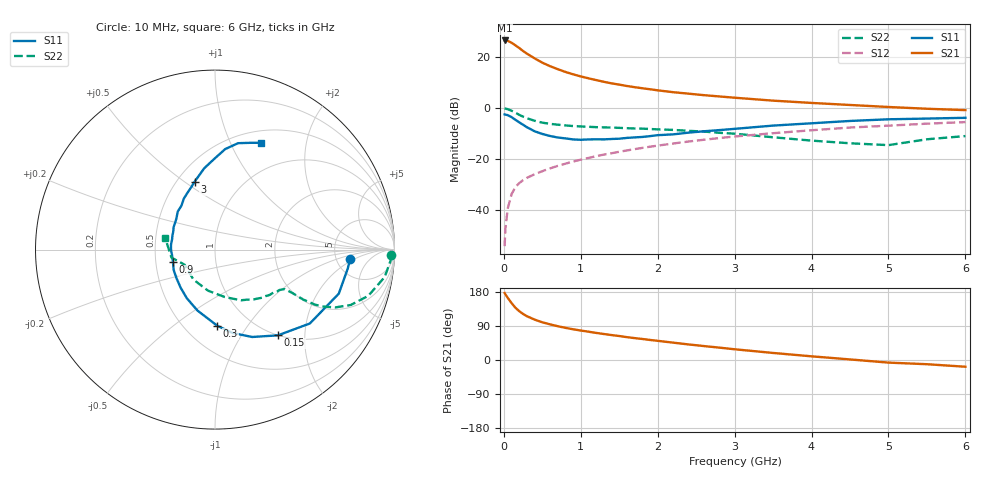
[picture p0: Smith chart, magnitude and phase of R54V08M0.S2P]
! SIEMENS Small Signal Semiconductors
! BFR183
! Si NPN RF Bipolar Junction Transistor in SOT23
! VCE = 4 V  IC = 8 mA
! Common Emitter S-Parameters:  May  1996
# GHz  S  MA  R  50
!  f  S11  S21  S12  S22
! GHz  MAG  ANG  MAG  ANG  MAG  ANG  MAG  ANG
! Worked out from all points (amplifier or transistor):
!   36 points, 10 MHz to 6 GHz, reference 50 ohm
!   highest |S21| = 26.5 dB at 10 MHz (marker M1)
!   |S21| within 3 dB of that: start of sweep to 201.7 MHz
!   unconditionally stable (mu >= 1): 862.4 MHz to 2.515 GHz
!   at 250 MHz: K = 0.55, MSG = 25.3 dB, |S12| = -28.2 dB
!   at 1.4 GHz: K = 1.06, MAG = 12.2 dB, |S12| = -17.6 dB
!   at 6 GHz: K = 0.88, MSG = 2.3 dB, |S12| = -5.4 dB
!   lowest NFmin = 1.30 dB at 450 MHz
!   S11 on the Smith chart (normalised r, x): 10 MHz: 6.74, -1.65; 150 MHz: 1.00, -1.47; 300 MHz: 0.71, -0.73; 900 MHz: 0.62, -0.09; 3 GHz: 0.61, +0.55; 6 GHz: 0.64, +1.32
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0.01  0.7548 -4.0  21.14 176.8  0.002 84.1  0.9835 -1.8
0.02  0.7472 -8.1  21.07 173.3  0.0043 84.2  0.9797 -3.7
0.05  0.7321 -19.6  20.82 164.3  0.0108 81.9  0.9576 -9.2
0.1  0.6698 -37.9  19.09 150.4  0.0207 73.6  0.8918 -16.8
0.15  0.5927 -53.7  16.99 138.0  0.0286 67.3  0.8168 -22.2
0.2  0.529 -67.0  15.03 128.9  0.0342 64.0  0.743 -25.7
0.25  0.4741 -78.2  13.14 121.5  0.0391 62.0  0.6829 -27.7
0.3  0.4243 -88.3  11.66 115.5  0.0435 61.1  0.6373 -28.8
0.4  0.3535 -106.0  9.437 106.6  0.051 60.8  0.567 -29.5
0.5  0.3134 -120.0  7.775 99.5  0.0586 61.5  0.5211 -29.4
0.6  0.286 -132.0  6.641 94.1  0.0664 61.8  0.4945 -29.3
0.7  0.267 -143.6  5.808 89.2  0.0744 62.3  0.4758 -29.4
0.9  0.2447 -163.1  4.601 81.1  0.0905 63.3  0.4477 -29.5
1.1  0.2449 -179.1  3.843 74.7  0.1065 63.5  0.4326 -31.0
1.3  0.2455 167.6  3.284 68.6  0.1237 63.2  0.4213 -32.6
1.6  0.2625 151.4  2.718 60.3  0.1492 62.1  0.4059 -36.2
2.2  0.3077 127.5  2.057 45.8  0.2036 58.0  0.3762 -45.4
3  0.3946 106.8  1.603 28.3  0.2794 50.1  0.3173 -62.9
3.5  0.4566 97.6  1.405 18.6  0.3242 44.2  0.2699 -78.3
4.5  0.5629 84.2  1.156 1.5  0.4186 32.1  0.2059 -125.5
5.5  0.6266 71.7  0.975 -11.1  0.4984 20.1  0.2467 -169.6
6  0.6487 66.5  0.917 -17.8  0.5352 12.3  0.2851 166.8
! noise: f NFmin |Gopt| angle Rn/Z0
0.45  1.3  0.17  43  0.21
0.9  1.35  0.21  115  0.2
1.8  2.05  0.33  -177  0.14
